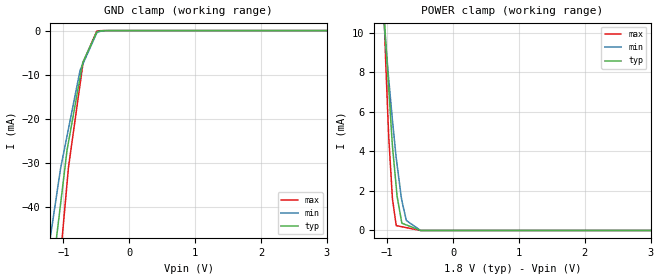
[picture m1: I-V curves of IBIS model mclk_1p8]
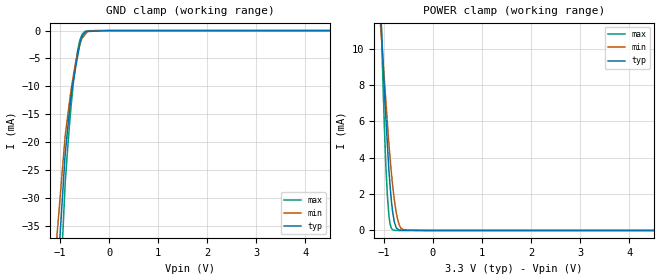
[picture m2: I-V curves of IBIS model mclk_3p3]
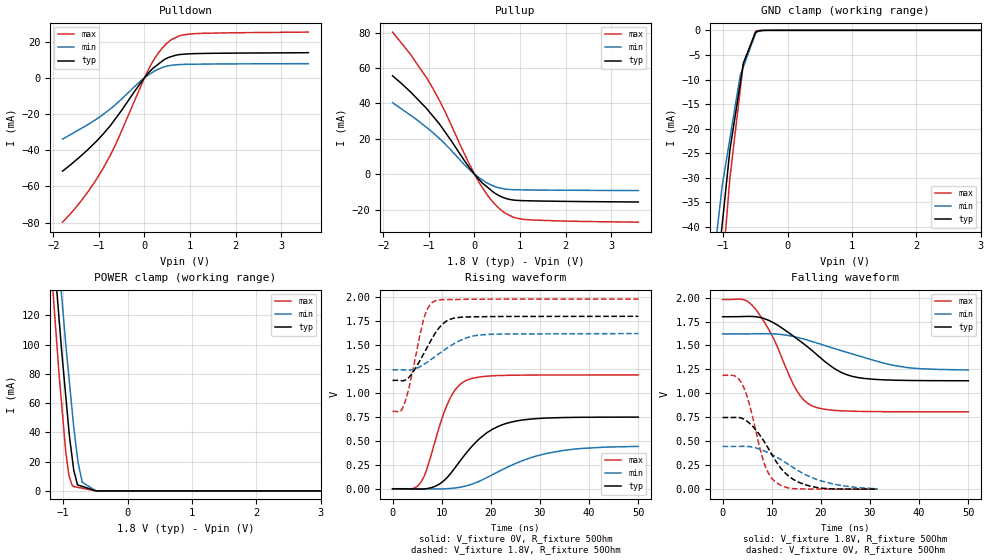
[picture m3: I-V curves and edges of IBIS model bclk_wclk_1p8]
|Texas Instruments Incorporated
| Low-Power Stereo Codec with 6 Inputs, 6 Outputs, Integrated Headphone/Speaker
| Amps, 3D Effects
| Marketing part#   Digital Voltage Range   Package-type   #pins
| TLV320AIC31IRHBR   1.1V-3.6V   QFN   32
| TLV320AIC31IRHBRG4  1.1V-3.6V   QFN   32
| TLV320AIC31IRHBT   1.1V-3.6V   QFN   32
| TLV320AIC31IRHBTG4  1.1V-3.6V   QFN   32
[IBIS Ver]   3.2
[File name]   tlv320aic31.ibs
|SIMDE Ver   V3.0 - 201101 - RHL4 - Build 457
[File Rev]   1.1
[Date]   9/21/2011
[Source]
| Texas Instruments Incorporated.
| Analog-eLab Design Center, HPA
| 12500 TI Blvd
| Dallas, TX -75243
| e-mail: elab_scm_ibis@list.ti.com
[Notes]   Revision History:
| Rev 1.0: 8/29/2011
| - Initial version of the model
| - Model generated from simulations in TISPICE
| - Model matched to SPICE simulation
| - C_comp although listed in numerical order of value are
|   obtained from varying PVT conditions. For PVT conditions for
|   each specific value refer the buffer description under
|   respective [Model]. IBIS model user is responsible for using
|   appropriate C_comp to simulate for Signal Integrity.
| - Model names with a trailing _1p8 contains the model for
|   1.8V [1.62V and 1.98V].Model names with a trailing _3p3
|   contains the model for 3.3V [3.0V and 3.6V].
| Rev 1.1: 9/21/2011
| - Updated the C_Comp values by removing bondpad from the netlist
[Disclaimer]
| This model is designed as an aid for customers of Texas Instruments.
| TI and its licensors and suppliers make no warranties, either expressed
| or implied, with respect to this  model, including the warranties of
| merchantability or fitness for a particular purpose. The model is
| provided solely on an "as is" basis. The entire risk as to its quality
| and performance is with the customer.
[Copyright]
 (C) Copyright 2011 Texas Instruments Incorporated.All rights reserved.
|   TLV320AIC31
[Component]   TLV320AIC31
[Manufacturer]   TI
[Package]   |32 QFN -  RHB package
|   typ   min   max
R_pkg   0.07718   0.03258   0.11084
L_pkg   1.34741nH   0.76736nH   1.81874nH
C_pkg   0.19486pF   0.16263pF   0.25079pF
[Pin]  signal_name   model_name   R_pin   L_pin   C_pin
1   MCLK   MCLK   0.10980   1.80738nH  0.20351pF
2   BCLK   BCLK_WCLK   0.04834   1.27894nH  0.25079pF
3   WCLK   BCLK_WCLK   0.04153   1.05595nH  0.22423pF
4   DIN   DIN   0.07341   1.17495nH  0.17505pF
5   DOUT   DOUT   0.06543   1.04328nH  0.16455pF
6   DVSS   GND   0.06617   1.05558nH  0.16473pF
7   IOVDD   POWER   0.07422   1.18976nH  0.17262pF
8   SCL   SCL   0.09445   1.54209nH  0.17632pF
9   SDA   SDA   0.10381   1.70349nH  0.18628pF
10   IN1LP   TERM   0.09706   1.57875nH  0.19190pF
11   IN1LM   TERM   0.11084   1.81874nH  0.21129pF
12   IN1RP   TERM   0.09921   1.61505nH  0.20474pF
13   IN1RM   TERM   0.09378   1.51996nH  0.19828pF
14   IN2L   TERM   0.09457   1.53226nH  0.19911pF
15   MICBIAS   TERM   0.10123   1.64737nH  0.20366pF
16   IN2R   TERM   0.11073   1.81870nH  0.19581pF
17   AVSS1   GND   0.10587   1.73309nH  0.18653pF
18   DRVDD   POWER   0.08549   1.37555nH  0.18063pF
19   HPLOUT   TERM   0.04394   1.15760nH  0.22090pF
20   HPLCOM   TERM   0.03761   0.93514nH  0.20874pF
21   DRVSS   GND   0.03475   0.83845nH  0.19402pF
22   HPRCOM   TERM   0.03258   0.76736nH  0.18547pF
23   HPROUT   TERM   0.03636   0.90542nH  0.19865pF
24   DRVDD   POWER   0.04412   1.17412nH  0.20375pF
25   AVDD   POWER   0.04645   1.25584nH  0.20175pF
26   AVSS2   GND   0.04847   1.29980nH  0.22244pF
27   LEFT_LOP   TERM   0.09345   1.51004nH  0.19823pF
28   LEFT_LOM   TERM   0.07850   1.25496nH  0.18383pF
29   RIGHT_LOP   TERM   0.06952   1.10594nH  0.17081pF
30   RIGHT_LOM   TERM   0.07016   1.11884nH  0.16699pF
31   _RESET   RESET   0.06890   1.09832nH  0.16263pF
32   DVDD   POWER   0.10602   1.74027nH  0.18605pF
33   THERMAL_PAD   NC   0.00085   0.24617nH  2.29047pF
[Pin Mapping]  pulldown_ref pullup_ref gnd_clamp_ref power_clamp_ref
1   GNDBUS3   PWRBUS1
2   GNDBUS3   PWRBUS1
3   GNDBUS3   PWRBUS1
4   GNDBUS3   PWRBUS1
5   GNDBUS3   PWRBUS1
6   GNDBUS1   NC
7   NC   PWRBUS1
8   GNDBUS3   PWRBUS1
9   GNDBUS3   PWRBUS1
10   GNDBUS3   PWRBUS2
11   GNDBUS3   PWRBUS2
12   GNDBUS3   PWRBUS2
13   GNDBUS3   PWRBUS2
14   GNDBUS3   PWRBUS2
15   GNDBUS3   PWRBUS2
16   GNDBUS3   PWRBUS2
17   GNDBUS2   NC
18   NC   PWRBUS2
19   GNDBUS3   PWRBUS2
20   GNDBUS3   PWRBUS2
21   GNDBUS3   NC
22   GNDBUS3   PWRBUS2
23   GNDBUS3   PWRBUS2
24   NC   PWRBUS2
25   NC   PWRBUS3
26   GNDBUS4   NC
27   GNDBUS3   PWRBUS3
28   GNDBUS3   PWRBUS3
29   GNDBUS3   PWRBUS3
30   GNDBUS3   PWRBUS3
31   GNDBUS3   PWRBUS1
32   NC   PWRBUS4
33   NC   NC
|   Model Selectors
[Model Selector] MCLK
mclk_1p8   1.8V digital input
mclk_3p3   3.3V digital input
[Model Selector] BCLK_WCLK
bclk_wclk_1p8   1.8V digital I/O
bclk_wclk_3p3   3.3V digital I/O
[Model Selector] DIN
din_1p8   1.8V digital input
din_3p3   3.3V digital input
[Model Selector] DOUT
dout_1p8   1.8V digital output
dout_3p3   3.3V digital output
[Model Selector] RESET
reset_1p8   1.8V digital input
reset_3p3   3.3V digital input
[Model Selector] SCL
scl_1p8   1.8V digital input
scl_3p3   3.3V digital input
[Model Selector] SDA
sda_1p8   1.8V digital open_drain
sda_3p3   3.3V digital open_drain
[Model Selector] TERM
term_1p8   1.8V nominal termination
term_3p3   3.3V nominal termination
[Model] term_1p8
Model_type Terminator
C_comp   1.0e-20F  1.0e-20F  1.0e-20F
|   typ   min   max
[Voltage Range]   1.8V   1.62V   1.98V
[POWER Clamp Reference]   1.8V   1.62V   1.98V
[GND Clamp Reference]   0V   0V   0V
|Ambient Temperature   25   85   -40
|Junction Temperature
[Temperature Range]   26   86   -40
[Model] term_3p3
Model_type Terminator
C_comp   1.0e-20F  1.0e-20F  1.0e-20F
|   typ   min   max
[Voltage Range]   3.3V   3.0V   3.6V
[POWER Clamp Reference]   3.3V   3.0V   3.6V
[GND Clamp Reference]   0V   0V   0V
|Ambient Temperature   25   85   -40
|Junction Temperature
[Temperature Range]   26   86   -40
| Models and submodels in the file (16): mclk_1p8 (Input), mclk_3p3 (Input), bclk_wclk_1p8 (I/O), bclk_wclk_3p3 (I/O), din_1p8 (Input), din_3p3 (Input), dout_1p8 (Output), dout_3p3 (Output), reset_1p8 (Input), reset_3p3 (Input), scl_1p8 (Input), scl_3p3 (Input), sda_1p8 (Open_drain), sda_3p3 (Open_drain), term_1p8 (Terminator), term_3p3 (Terminator)
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|   mclk_1p8 Model
[Model]   mclk_1p8
Model_type   Input
Vinl = 0.54
Vinh = 1.26
|   typ   min   max
|   (nom PVT)   (fast PVT)   (slow PVT)
|C_comp from frequency sweep method (F=50MHz)
|Average
C_comp   6.483e-12   6.453e-12   6.553e-12
|C_comp from LC tank measurement(L=1nH)
|Average
|Resonant Frequency(Hz)   2.070e+09   2.090e+09   2.060e+09
|C_comp   5.917e-12   5.805e-12   5.975e-12
| Where nom  PVT is Nominal Process, 1.8V, 26C
|   Fast PVT is Strong Process,  1.98V, -40C
|   Slow PVT is Weak Process,   1.62V, 86C
[Model Spec]
|Subparameter   typ   min   max
Vinl   0.54   0.486   0.594
Vinh   1.26   1.134   1.386
[Voltage Range]   1.8   1.62   1.98
|Ambient Temperature   25   85   -40
|Junction Temperature
[Temperature Range]   26   86   -40
[Power Clamp Reference]   1.8   1.62   1.98
[GND Clamp Reference]   0   0   0
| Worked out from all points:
|   GND clamp passes 1 mA (typ) near -0.52 V on its own axis
|   POWER clamp passes 1 mA (typ) near -0.81 V on its own axis
[GND Clamp]
|   Voltage   I(typ)   I(min)   I(max)
-1.8V     -248.6mA   -142.9mA   -345.7mA
-1.215V   -60.5mA    -48.36mA   -81.14mA
-1.178V   -55.92mA   -44.66mA   -73.2mA
-1.043V   -39.19mA   -31.17mA   -50.81mA
-945mV    -27.02mA   -23.8mA    -34.49mA
-922.7mV  -25.17mA   -22.13mA   -30.84mA
-746.8mV  -10.54mA   -8.95mA    -12.06mA
-707.4mV  -7.264mA   -7.634mA   -7.852mA
-700.9mV  -7.053mA   -7.418mA   -7.16mA
-495mV    -338.9uA   -547.1uA   -147.5uA
-306.2mV  -2.612uA   -6.398uA   -288.4nA
3.6V      0A         0A         0A
[POWER Clamp]
|   Voltage   I(typ)   I(min)   I(max)
-1.8V     58.58mA    42.75mA    96.1mA
-1.073V   12.51mA    11.5mA     13.37mA
-1.033V   10.12mA    9.9mA      9.534mA
-1.022V   9.52mA     9.438mA    8.427mA
-976.1mV  7.154mA    7.627mA    4.701mA
-920.7mV  4.294mA    5.584mA    1.615mA
-863.3mV  2.217mA    3.671mA    247uA
-849.6mV  1.724mA    3.318mA    237.9uA
-777.6mV  369.1uA    1.512mA    189.6uA
-709.6mV  280.2uA    505.5uA    143.9uA
-494.1mV  18.66nA    1.306uA    0A
3.6V      0A         0A         0A
|   mclk_3p3 Model
[Model]   mclk_3p3
Model_type   Input
Vinl = 0.99
Vinh = 2.31
|   typ   min   max
|   (nom PVT)   (fast PVT)   (slow PVT)
|C_comp from frequency sweep method (F=50MHz)
|Average
C_comp   6.042e-12   5.998e-12   6.135e-12
|C_comp from LC tank measurement(L=1nH)
|Average
|Resonant Frequency(Hz)   2.150e+09   2.170e+09   2.140e+09
|C_comp   5.485e-12   5.385e-12   5.537e-12
| Where nom  PVT is Nominal Process, 3.3V, 26C
|   Fast PVT is Strong Process,  3.6V, -40C
|   Slow PVT is Weak Process,   3V, 86C
[Model Spec]
|Subparameter   typ   min   max
Vinl   0.99   0.9   1.08
Vinh   2.31   2.1   2.52
[Voltage Range]   3.3   3   3.6
|Ambient Temperature   25   85   -40
|Junction Temperature
[Temperature Range]   26   86   -40
[Power Clamp Reference]   3.3   3   3.6
[GND Clamp Reference]   0   0   0
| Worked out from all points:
|   GND clamp passes 1 mA (typ) near -0.55 V on its own axis
|   POWER clamp passes 1 mA (typ) near -0.82 V on its own axis
[GND Clamp]
|   Voltage   I(typ)   I(min)   I(max)
-3.3V     -1.384A    -1.199A    -1.638A
-1.451V   -99.45mA   -78.32mA   -132.3mA
-897.6mV  -22.27mA   -18.95mA   -27.54mA
-842.4mV  -17.31mA   -15.11mA   -20.63mA
-792mV    -13.07mA   -11.62mA   -15.13mA
-745.8mV  -9.711mA   -8.96mA    -10.77mA
-691.2mV  -7.004mA   -6.098mA   -6.475mA
-601.2mV  -2.542mA   -2.645mA   -1.857mA
-554.4mV  -1.128mA   -1.419mA   -707.6uA
-500.4mV  -468.1uA   -819.4uA   -172.4uA
-285mV    -101.7uA   -3.563uA   -12.71uA
6.6V      0A         0A         0A
[POWER Clamp]
|   Voltage   I(typ)   I(min)   I(max)
-3.3V     157.9mA    110.4mA    274.6mA
-1.089V   13.36mA    12.1mA     15.18mA
-1.037V   10.41mA    10.1mA     9.822mA
-993.6mV  7.977mA    8.451mA    6.026mA
-961.2mV  6.3mA      7.213mA    3.694mA
-928.8mV  4.786mA    5.974mA    1.956mA
-874.8mV  2.533mA    4.048mA    387.6uA
-820.8mV  1.031mA    2.477mA    39.19uA
-785.4mV  455.6uA    1.675mA    15.66uA
-717mV    84.01uA    584.6uA    1.359uA
-591mV    14.18uA    23.34uA    0A
6.6V      0A         0A         0A
|   bclk_wclk_1p8 Model
[Model]   bclk_wclk_1p8
Model_type   I/O
Polarity   Non-Inverting
Enable   Active-Low
Vinl = 0.54
Vinh = 1.26
Vmeas = 0.9
Vref = 0.9
Cref = 10pF
Rref = 50
|   typ   min   max
|   (nom PVT)   (fast PVT)   (slow PVT)
|C_comp from frequency sweep method (F=25MHz)
|C_comp   1.245e-11   1.140e-11   1.295e-11
|ON state : BUFFER OUTPUT TURNED HIGH
|C_comp   1.612e-11   1.418e-11   1.698e-11
|OFF state: BUFFER IN HIGH IMPEDANCE
|C_comp   8.770e-12   8.611e-12   8.919e-12
|C_comp from LC tank measurement(L=1nH)
|Average
|Resonant Frequency(Hz)   2.075e+09   2.085e+09   2.065e+09
C_comp   5.897e-12   5.841e-12   5.951e-12
|ON state : BUFFER OUTPUT TURNED HIGH
|Resonant Frequency(Hz)   2.030e+09   2.040e+09   2.030e+09
|C_comp   6.153e-12   6.093e-12   6.153e-12
|OFF state: BUFFER IN HIGH IMPEDANCE
|Resonant Frequency(Hz)   2.120e+09   2.130e+09   2.100e+09
|C_comp   5.642e-12   5.589e-12   5.750e-12
| Where nom  PVT is Nominal Process, 1.8V, 26C
|   Fast PVT is Strong Process,  1.98V, -40C
|   Slow PVT is Weak Process,   1.62V, 86C
[Model Spec]
|Subparameter   typ   min   max
Vinl   0.54   0.486   0.594
Vinh   1.26   1.134   1.386
[Voltage Range]   1.8   1.62   1.98
|Ambient Temperature   25   85   -40
|Junction Temperature
[Temperature Range]   26   86   -40
[Pullup Reference]   1.8   1.62   1.98
[Pulldown Reference]   0   0   0
[Power Clamp Reference]   1.8   1.62   1.98
[GND Clamp Reference]   0   0   0
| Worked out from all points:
|   slope of the pulldown table from 0 to 0.27 V, typ, clamps not added: 39.2 ohm
|   slope of the pullup table from 0 to 0.27 V, typ, clamps not added: 38.2 ohm
|   GND clamp passes 1 mA (typ) near -0.51 V on its own axis
|   POWER clamp passes 1 mA (typ) near -0.56 V on its own axis
|   falling waveform, V_fixture 1.8V, R_fixture 50Ohm: 20-80 % time 10ns typ, 14.5ns min, 6.46ns max; typ from 1.8 V to 1.13 V
|   rising waveform, V_fixture 0V, R_fixture 50Ohm: 20-80 % time 7.95ns typ, 12.1ns min, 4.6ns max; typ from 0 V to 0.748 V
|   rising waveform, V_fixture 1.8V, R_fixture 50Ohm: 20-80 % time 4.51ns typ, 6.66ns min, 2.94ns max; typ from 1.13 V to 1.8 V
|   falling waveform, V_fixture 0V, R_fixture 50Ohm: 20-80 % time 6.05ns typ, 9.53ns min, 3.61ns max; typ from 0.748 V to 0.001 V
[Pulldown]
|   Voltage   I(typ)   I(min)   I(max)
-1.8V     -51.54mA   -33.88mA   -79.76mA
-1.602V   -47.56mA   -31.03mA   -74.43mA
-1.243V   -39.65mA   -25.85mA   -63.03mA
-910.8mV  -31.15mA   -20.25mA   -50.1mA
-631.6mV  -22.38mA   -14.64mA   -36.66mA
-72mV     -2.397mA   -1.514mA   -4.136mA
128.7mV   3.784mA    2.245mA    6.619mA
344.5mV   8.331mA    5.151mA    15.06mA
568.3mV   11.56mA    6.838mA    20.63mA
756.4mV   12.78mA    7.283mA    23.08mA
1.109V    13.36mA    7.516mA    24.38mA
3.6V      13.88mA    7.817mA    25.25mA
[GND Clamp]
|   Voltage   I(typ)   I(min)   I(max)
-1.8V     -232.8mA   -141.8mA   -328.8mA
-1.129V   -53.85mA   -44.78mA   -70.72mA
-1.016V   -39.58mA   -31.71mA   -49.39mA
-896.9mV  -24.56mA   -22.17mA   -30.29mA
-894.6mV  -24.3mA    -21.98mA   -29.96mA
-735.5mV  -10.87mA   -9.202mA   -12.19mA
-689mV    -6.946mA   -7.542mA   -6.997mA
-685.8mV  -6.672mA   -7.426mA   -6.883mA
-495mV    -374.3uA   -603.1uA   -162.8uA
-424.4mV  -64.4uA    -133.7uA   -19.47uA
-306.2mV  -2.877uA   -7.045uA   -317.7nA
3.6V      0A         0A         0A
[Pullup]
|   Voltage   I(typ)   I(min)   I(max)
-1.8V     55.63mA    40.44mA    80.35mA
-1.41V    46.62mA    33.39mA    67.87mA
-980.1mV  34.88mA    24.96mA    51.38mA
-631.6mV  23.33mA    16.68mA    34.57mA
-140.6mV  4.737mA    3.33mA     7.104mA
53.46mV   -1.611mA   -1.125mA   -2.516mA
180mV     -5.162mA   -3.334mA   -7.856mA
348.5mV   -8.737mA   -5.893mA   -14.02mA
601.9mV   -12.89mA   -8.07mA    -20.69mA
845.5mV   -14.6mA    -8.797mA   -24.33mA
1.109V    -15.01mA   -8.899mA   -25.65mA
3.6V      -15.74mA   -9.284mA   -27.16mA
[POWER Clamp]
|   Voltage   I(typ)   I(min)   I(max)
-1.8V     544.9mA    560.9mA    549.9mA
-1.204V   194.6mA    228.6mA    164.2mA
-1.115V   145.6mA    180.3mA    110.3mA
-1.063V   117.6mA    153.9mA    79.5mA
-1.022V   95.22mA    132.8mA    58.63mA
-962.3mV  66.12mA    101.8mA    27.94mA
-910.8mV  41.2mA     77.96mA    10.68mA
-837.5mV  14.93mA    44.52mA    3.047mA
-777.6mV  4.167mA    22.59mA    2.521mA
-703.1mV  3.089mA    5.883mA    1.867mA
-494.1mV  76.44uA    107.5uA    41.21uA
3.6V      0A         0A         0A
[Ramp]
R_load = 50
|   typ   min   max
dV/dt_r   0.44863/7.93386e-09   0.26526/1.20115e-08   0.712746/4.5894e-09
dV/dt_f   0.400991/1.00322e-08   0.225254/1.45075e-08   0.703437/6.45624e-09
[Falling Waveform]
V_fixture = 1.8V
V_fixture_min = 1.62V
V_fixture_max = 1.98V
R_fixture = 50Ohm
|   Time   V(typ)   V(min)   V(max)
0s        1.8V       1.62V      1.98V
4.235ns   1.802V     1.62V      1.979V
6.555ns   1.801V     1.622V     1.889V
10.33ns   1.738V     1.621V     1.577V
15.04ns   1.574V     1.587V     1.034V
18.2ns    1.447V     1.541V     869.2mV
23.41ns   1.239V     1.457V     820.3mV
27.53ns   1.165V     1.394V     812.2mV
37.69ns   1.135V     1.269V     808.1mV
50ns      1.132V     1.245V     807.6mV
[Rising Waveform]
V_fixture = 0V
V_fixture_min = 0V
V_fixture_max = 0V
R_fixture = 50Ohm
|   Time   V(typ)   V(min)   V(max)
0s        914.4pV    5.585nV    571.3pV
4.005ns   -2.558mV   -396uV     -551.5uV
5.745ns   -3.339mV   -1.585mV   67.35mV
6.925ns   1.267mV    -2.151mV   196.9mV
11.27ns   125.9mV    1.048mV    896.1mV
14.95ns   370.4mV    29.74mV    1.13V
19.32ns   588.8mV    119.8mV    1.175V
24.85ns   704mV      260mV      1.185V
34.6ns    743.1mV    399.1mV    1.187V
50ns      747.7mV    442.1mV    1.188V
[Rising Waveform]
V_fixture = 1.8V
V_fixture_min = 1.62V
V_fixture_max = 1.98V
R_fixture = 50Ohm
|   Time   V(typ)   V(min)   V(max)
0s        1.131V     1.241V     807.5mV
1.5ns     1.129V     1.242V     806.8mV
2.33ns    1.13V      1.24V      874.9mV
3.56ns    1.176V     1.24V      1.103V
6.375ns   1.413V     1.298V     1.779V
7.49ns    1.519V     1.337V     1.91V
8.7ns     1.626V     1.382V     1.962V
11.33ns   1.76V      1.477V     1.975V
17.17ns   1.795V     1.601V     1.978V
50ns      1.8V       1.62V      1.98V
[Falling Waveform]
V_fixture = 0V
V_fixture_min = 0V
V_fixture_max = 0V
R_fixture = 50Ohm
|   Time   V(typ)   V(min)   V(max)
0s        748.1mV    446.3mV    1.188V
2.51ns    748.9mV    446.1mV    1.182V
4.02ns    738.2mV    447.1mV    1.092V
5.455ns   688.9mV    444.3mV    886.1mV
8.39ns    502.9mV    400.7mV    281.4mV
9.66ns    394.1mV    370.7mV    138.4mV
10.92ns   286.8mV    336.7mV    68.29mV
13.65ns   128.1mV    250mV      10.89mV
17.61ns   34.68mV    133mV      1.655mV
31.52ns   633.6uV    3.938mV    181.6uV
